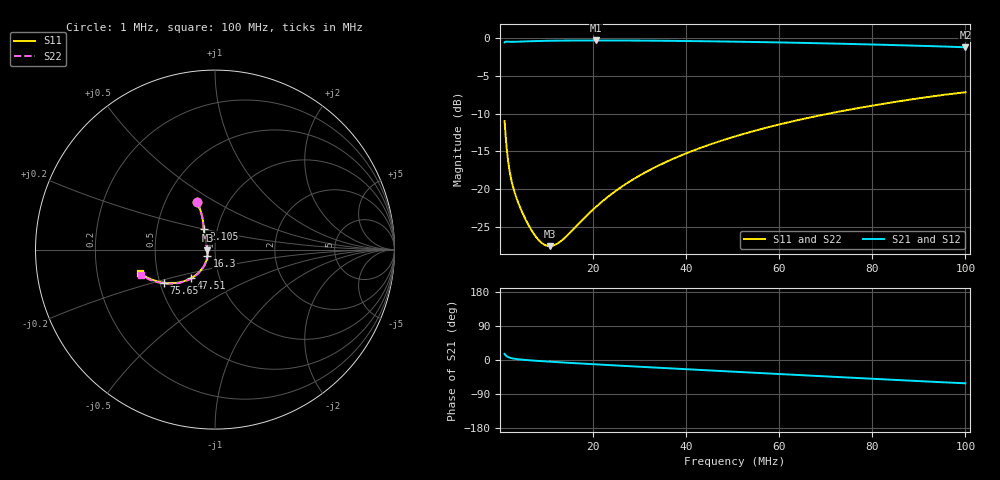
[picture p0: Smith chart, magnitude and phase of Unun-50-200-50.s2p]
! ListType=Log
!!Unun 2 Unun 50-200-50
# MHZ S RI R 50
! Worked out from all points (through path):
!   100 points, 1 MHz to 100 MHz, reference 50 ohm
!   highest |S21| = -0.36 dB at 20.57 MHz (marker M1); lowest = -1.3 dB at 100 MHz (marker M2)
!   group delay of S21, straight-line fit = 1.99 ns
!   lowest |S11| = -27.5 dB at 10.72 MHz (marker M3), VSWR 1.09, Z = 46 - j0.376 ohm
!   |S11| at or under -10 dB: start of sweep to 70.75 MHz
!   |S22| runs from -27.5 to -7.2 dB; largest |S21 - S12| = 0.0038
!   S11 on the Smith chart (normalised r, x): 1 MHz: 0.72, +0.41; 2.105 MHz: 0.86, +0.20; 16.3 MHz: 0.92, -0.07; 47.51 MHz: 0.73, -0.24; 75.65 MHz: 0.53, -0.22; 100 MHz: 0.40, -0.13
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1  -0.101 0.2636  0.8974 0.2564  0.8975 0.2563  -0.101 0.2635
1.261857  -0.0768 0.2036  0.9216 0.1946  0.9216 0.1946  -0.0768 0.2035
1.519911  -0.0682 0.1643  0.93 0.1536  0.93 0.1536  -0.0682 0.1642
2.104904  -0.0627 0.1146  0.9352 0.1  0.9353 0.1  -0.0627 0.1146
2.782559  -0.0601 0.0857  0.9375 0.0667  0.9375 0.0667  -0.0601 0.0857
3.67838  -0.0567 0.0641  0.9405 0.0392  0.9405 0.0392  -0.0568 0.064
6.135907  -0.0487 0.0317  0.9474 -0.00893  0.9474 -0.00893  -0.0487 0.0316
8.497534  -0.0442 0.0115  0.9508 -0.044  0.9508 -0.044  -0.0442 0.0115
9.7701  -0.0427 0.00232  0.9517 -0.0612  0.9517 -0.0612  -0.0427 0.00225
10.72267  -0.042 -0.00408  0.9519 -0.0736  0.952 -0.0737  -0.042 -0.00417
12.9155  -0.0414 -0.0179  0.9514 -0.1012  0.9515 -0.1012  -0.0413 -0.018
16.29751  -0.0427 -0.0373  0.9482 -0.1417  0.9482 -0.1417  -0.0425 -0.0374
17.8865  -0.0442 -0.0458  0.9457 -0.1602  0.9457 -0.1602  -0.044 -0.046
20.56512  -0.0477 -0.0595  0.9404 -0.1906  0.9404 -0.1906  -0.0474 -0.0597
27.18588  -0.0613 -0.0904  0.9218 -0.2626  0.9217 -0.2627  -0.0608 -0.0907
34.30469  -0.0822 -0.1191  0.8942 -0.3358  0.8942 -0.3358  -0.0814 -0.1196
47.5081  -0.1346 -0.16  0.8257 -0.4595  0.8258 -0.4596  -0.1332 -0.1611
52.14008  -0.1564 -0.1702  0.797 -0.4989  0.7971 -0.499  -0.1547 -0.1717
68.92612  -0.245 -0.1871  0.6766 -0.6223  0.6767 -0.6224  -0.2425 -0.1903
75.64633  -0.2829 -0.1847  0.6225 -0.6628  0.6225 -0.6627  -0.2802 -0.1887
86.9749  -0.3472 -0.1689  0.5261 -0.7185  0.5262 -0.7185  -0.3444 -0.1746
100  -0.4163 -0.132  0.4138 -0.7594  0.4166 -0.762  -0.4148 -0.1413
